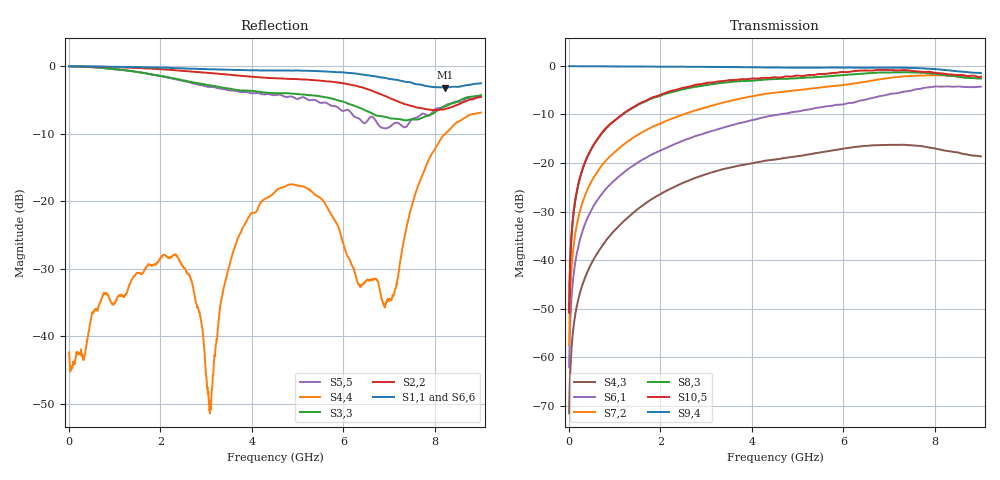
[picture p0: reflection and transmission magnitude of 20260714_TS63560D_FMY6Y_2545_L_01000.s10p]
# GHz S DB R 50
! CMT, SN0916, 25263762, 26.7.0
! Date: 15.07.2026 13:37:25
! Data: Format
! Freq S1.1:dB/Ang S1.2:dB/Ang S1.3:dB/Ang S1.4:dB/Ang S1.5:dB/Ang S1.6:dB/Ang S1.7:dB/Ang S1.8:dB/Ang S1.9:dB/Ang S1.10:dB/Ang
!  S2.1:dB/Ang S2.2:dB/Ang S2.3:dB/Ang S2.4:dB/Ang S2.5:dB/Ang S2.6:dB/Ang S2.7:dB/Ang S2.8:dB/Ang S2.9:dB/Ang S2.10:dB/Ang
!  S3.1:dB/Ang S3.2:dB/Ang S3.3:dB/Ang S3.4:dB/Ang S3.5:dB/Ang S3.6:dB/Ang S3.7:dB/Ang S3.8:dB/Ang S3.9:dB/Ang S3.10:dB/Ang
!  S4.1:dB/Ang S4.2:dB/Ang S4.3:dB/Ang S4.4:dB/Ang S4.5:dB/Ang S4.6:dB/Ang S4.7:dB/Ang S4.8:dB/Ang S4.9:dB/Ang S4.10:dB/Ang
!  S5.1:dB/Ang S5.2:dB/Ang S5.3:dB/Ang S5.4:dB/Ang S5.5:dB/Ang S5.6:dB/Ang S5.7:dB/Ang S5.8:dB/Ang S5.9:dB/Ang S5.10:dB/Ang
!  S6.1:dB/Ang S6.2:dB/Ang S6.3:dB/Ang S6.4:dB/Ang S6.5:dB/Ang S6.6:dB/Ang S6.7:dB/Ang S6.8:dB/Ang S6.9:dB/Ang S6.10:dB/Ang
!  S7.1:dB/Ang S7.2:dB/Ang S7.3:dB/Ang S7.4:dB/Ang S7.5:dB/Ang S7.6:dB/Ang S7.7:dB/Ang S7.8:dB/Ang S7.9:dB/Ang S7.10:dB/Ang
!  S8.1:dB/Ang S8.2:dB/Ang S8.3:dB/Ang S8.4:dB/Ang S8.5:dB/Ang S8.6:dB/Ang S8.7:dB/Ang S8.8:dB/Ang S8.9:dB/Ang S8.10:dB/Ang
!  S9.1:dB/Ang S9.2:dB/Ang S9.3:dB/Ang S9.4:dB/Ang S9.5:dB/Ang S9.6:dB/Ang S9.7:dB/Ang S9.8:dB/Ang S9.9:dB/Ang S9.10:dB/Ang
!  S10.1:dB/Ang S10.2:dB/Ang S10.3:dB/Ang S10.4:dB/Ang S10.5:dB/Ang S10.6:dB/Ang S10.7:dB/Ang S10.8:dB/Ang S10.9:dB/Ang S10.10:dB/Ang
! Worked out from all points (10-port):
!   2001 points, 10 MHz to 9 GHz, reference 50 ohm
!   strongest paths, dB at 10 MHz, 2.257 GHz, 4.505 GHz, 6.753 GHz, 9 GHz:
!     S9,4: -0.1, -0.2, -0.4, -0.4, -1.5
!     S10,5: -50.8, -5.1, -2.4, -0.8, -2.2
!     S8,3: -50.7, -5.4, -2.7, -1.4, -2.6
!     S7,2: -57.4, -10.9, -5.5, -2.8, -2.6
!     S6,1: -62.1, -16.4, -10.2, -6.3, -4.3
!     S4,3: -71.5, -25.1, -19.3, -16.3, -18.6
!   lowest |S11| = -3.2 dB at 8.213 GHz (marker M1), VSWR 5.54, Z = 11.1 - j23.5 ohm
!   |S11| at or under -10 dB: nowhere
